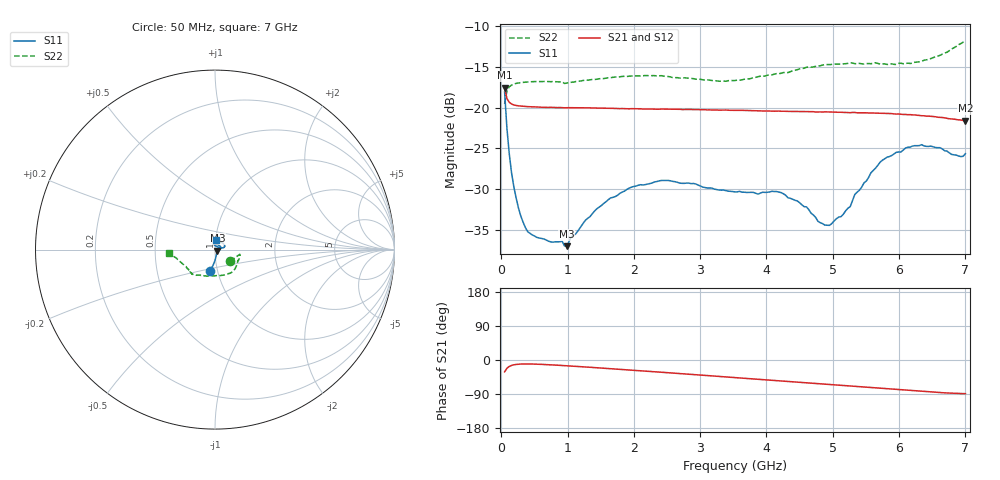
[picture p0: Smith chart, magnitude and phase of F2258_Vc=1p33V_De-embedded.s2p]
! Integrated Device Technology
! Corporate Headquarters
! 6024 Silver Creek Valley Road
! San Jose, CA 95138  USA
! Phone:  1-408-284-8200
! Toll Free:  1-800-223-1366
! Webpage:  http://www.idt.com/
! Timing and RF Division
! 515 Groton Road, Suite 102
! Westford, MA 01886-6024
! Device:  F2258
! Description: Voltage Variable RF Attenuator
! Frequency:  50.0 -  6000.00 MHz
! Package:  3x3 mm Thin QFN Plastic Package: 16 pin
! Ports:  2 RF, 2 DC
!  Pin  1  = NC
!  Pin  2  = NC
!  Pin  3  = RF2  = Port 2
!  Pin  4  = GND
!  Pin  5  = Vdd
!  Pin  6  = NC
!  Pin  7  = VCTRL
!  Pin  8  = NC
!  Pin  9  = GND
!  Pin 10  = RF1  = Port 1
!  Pin 11  = NC
!  Pin 12  = NC
!  Pin 13  = NC
!  Pin 14  = NC
!  Pin 15  = NC
!  Pin 16  = NC
! Vcntrl:  1.330 Volts
! Vdd:  +3.300 Volts
! Current:  1.167 mA
! Data:  The device was measured on a the F2258 evaluation board which has
!  individual transmission lines to the RF pins.  Data was collected
!  using a calibrated network analyzer.  The evaluation board was
!  de-embedded using a TRL calibration technique.
!  The reference plane is the edge of the package pin.
! Misc:  SN 10
!  Action Tracker AT0285
! Date Measured:  2014-12-10
! Date:  2016-01-13  MJV
! Note:
!  Integrated Device Technology supplies this data as a sample of measured
!  data at the package pin for this product.  Your particular data for this
!  product may vary.
!  Data was taken at 25 degrees C.
!  Integrated Device Technology reserves the right to change this data at anytime.
!Freq_(GHz)  S11M_(dB)  S11P_(deg)  S21M_(dB)  S21P_(deg)  S12M_(dB)  S12P_(deg)  S22M_(dB)  S22P_(deg)
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# GHz S dB R 50
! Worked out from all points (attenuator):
!   201 points, 50 MHz to 7 GHz, reference 50 ohm
!   highest |S21| = -17.55 dB at 50 MHz (marker M1); lowest = -21.6 dB at 7 GHz (marker M2)
!   lowest |S11| = -37.0 dB at 988.2 MHz (marker M3), VSWR 1.03, Z = 51.3 - j0.541 ohm
!   |S11| at or under -10 dB: start of sweep to end of sweep
!   |S22| runs from -19.5 to -11.8 dB; largest |S21 - S12| = 0.0012
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0.05  -18.08 -102.6  -17.55 -31.3  -17.60 -31.4  -19.55 -38.0
0.08475  -22.52 -94.0  -18.88 -21.8  -18.95 -21.9  -17.99 -18.4
0.15425  -27.98 -82.7  -19.55 -14.3  -19.63 -14.4  -17.24 -12.1
0.2585  -32.31 -68.0  -19.78 -11.1  -19.84 -11.1  -16.98 -11.0
0.328  -34.04 -58.2  -19.83 -10.5  -19.88 -10.5  -16.90 -11.9
0.467  -35.63 -42.5  -19.90 -10.6  -19.93 -10.6  -16.82 -14.0
0.98825  -37.01 -21.9  -20.01 -15.2  -20.05 -15.2  -16.99 -26.6
1.2315  -34.25 -8.7  -20.03 -17.9  -20.05 -17.9  -16.67 -32.0
1.6485  -31.09 0.8  -20.09 -23.0  -20.10 -23.0  -16.32 -40.9
2.37825  -29.00 19.8  -20.20 -31.8  -20.22 -31.8  -16.09 -56.4
3.525  -30.35 73.3  -20.34 -46.4  -20.36 -46.3  -16.67 -93.7
4.22  -30.43 99.4  -20.45 -55.3  -20.46 -55.3  -15.79 -117.8
4.7065  -33.17 86.0  -20.50 -61.5  -20.51 -61.4  -15.01 -127.5
4.88025  -34.42 68.8  -20.52 -63.8  -20.52 -63.7  -14.73 -129.7
5.1235  -33.38 40.7  -20.57 -66.7  -20.56 -66.8  -14.66 -132.5
5.2625  -32.17 26.4  -20.63 -68.4  -20.61 -68.5  -14.51 -133.9
5.332  -30.67 21.5  -20.60 -69.5  -20.62 -69.4  -14.61 -134.1
5.57525  -28.00 13.9  -20.66 -72.5  -20.68 -72.4  -14.62 -137.5
5.85325  -26.01 13.8  -20.73 -76.2  -20.74 -76.2  -14.66 -141.8
6.33975  -24.55 23.3  -21.00 -82.6  -21.00 -82.6  -14.31 -153.9
6.9305  -26.01 73.4  -21.52 -88.5  -21.50 -88.6  -12.14 -173.7
7  -25.66 83.8  -21.59 -88.8  -21.56 -88.9  -11.76 -176.3
